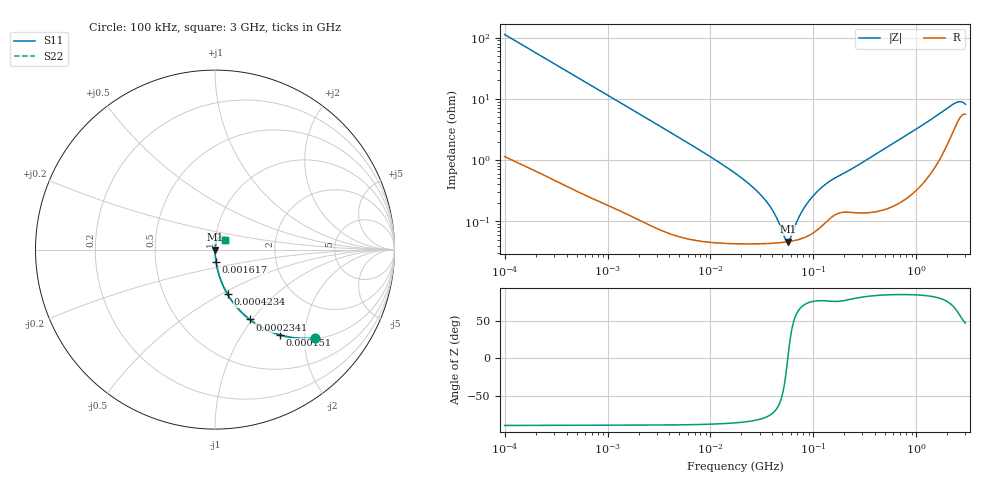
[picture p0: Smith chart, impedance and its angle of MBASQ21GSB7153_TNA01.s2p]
! MBASQ21GSB7153_TNA01  S-PARAMETER MODEL  ( Standard Model )
! Model Generated by TAIYO YUDEN Corporation (http://www.ty-top.com)
! Version 1.0
! TAIYO YUDEN Control No. 220601
! Copyright(c) 2013 TAIYO YUDEN CO.,LTD. All Rights Reserved.
! Product Description (link to TY-COMPAS)
! https://ds.yuden.co.jp/TYCOMPAS/or/detail?pn=MBASQ21GSB7153KTNA01&u=M
! Products Name : Multilayer Ceramic Capacitors
! Characteristics :
!  Capacitance : 0.015 [uF] , Rated Voltage : 250 [V] , TCC : X7R
!  Case Size : 2.0 x 1.25 / 0.079 x 0.049 [mm/inch] , Thickness : 1.25 / 0.049 [mm/inch]
!  (Conditions: Temperature = 25 [degC] , DC Bias Voltage = 0 [V])
! External Node Assignments :
!  1  o---| |---o  2
! GND o---------o GND
! Frequency Range : 100kHz  -  3GHz  [ 401 STEP ]
# MHZ S RI R 50
! Freq[MHz].  S11 Real  S11 Imag  S21 Real  S21 Imag  S12 Real  S12 Imag  S22 Real  S22 Imag
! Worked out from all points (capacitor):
!   401 points, 100 kHz to 3 GHz, reference 50 ohm
!   read as one part in series: C = 14.1 nF near 105.3 kHz
!   lowest |Z| = 46.2 mohm at 56.68 MHz (marker M1)
!   series resonance near 56.45 MHz, so ESL is about 560 pH
!   S11 on the Smith chart (normalised r, x): 100 kHz: 1.02, -2.26; 151 kHz: 1.02, -1.50; 234.1 kHz: 1.01, -0.97; 423.4 kHz: 1.01, -0.54; 1.617 MHz: 1.00, -0.14; 3 GHz: 1.11, +0.12
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0.1  0.5594 -0.4914  0.4406 0.4914  0.4406 0.4914  0.5594 -0.4914
0.151038  0.3608 -0.4748  0.6392 0.4748  0.6392 0.4748  0.3608 -0.4748
0.234079  0.1932 -0.3889  0.8068 0.3889  0.8068 0.3889  0.1932 -0.3889
0.423445  0.0704 -0.2493  0.9296 0.2493  0.9296 0.2493  0.0704 -0.2493
0.562235  0.0421 -0.1941  0.9579 0.1941  0.9579 0.1941  0.0421 -0.1941
1.61742  0.00629 -0.0707  0.9937 0.0707  0.9937 0.0707  0.00629 -0.0707
3.161081  0.00207 -0.0365  0.9979 0.0365  0.9979 0.0365  0.00207 -0.0365
17.7727  0.000462 -0.0059  0.9995 0.0059  0.9995 0.0059  0.000462 -0.0059
26.16047  0.000437 -0.0035  0.9996 0.0035  0.9996 0.0035  0.000437 -0.0035
34.73492  0.000434 -0.00209  0.9996 0.00209  0.9996 0.00209  0.000434 -0.00209
42.68829  0.00044 -0.00117  0.9996 0.00117  0.9996 0.00117  0.00044 -0.00117
53.83243  0.000456 -0.000197  0.9995 0.000197  0.9995 0.000197  0.000456 -0.000197
56.67997  0.000461 1.74e-05  0.9995 -1.74e-05  0.9995 -1.74e-05  0.000461 1.74e-05
59.67813  0.000468 0.000232  0.9995 -0.000232  0.9995 -0.000232  0.000468 0.000232
69.65816  0.000495 0.000884  0.9995 -0.000884  0.9995 -0.000884  0.000495 0.000884
77.22239  0.000522 0.00133  0.9995 -0.00133  0.9995 -0.00133  0.000522 0.00133
97.38194  0.000632 0.0024  0.9994 -0.0024  0.9994 -0.0024  0.000632 0.0024
143.341  0.0011 0.00433  0.9989 -0.00433  0.9989 -0.00433  0.0011 0.00433
547.5153  0.00193 0.0169  0.9981 -0.0169  0.9981 -0.0169  0.00193 0.0169
2259.438  0.0326 0.0715  0.9674 -0.0715  0.9674 -0.0715  0.0326 0.0715
2637.286  0.051 0.0688  0.949 -0.0688  0.949 -0.0688  0.051 0.0688
3000  0.0559 0.0532  0.9441 -0.0532  0.9441 -0.0532  0.0559 0.0532
